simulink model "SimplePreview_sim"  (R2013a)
settings: Solver=ode45  StartTime=0.0  StopTime=60  RelTol=1e-3
undefined symbols (not defined in the file or in its folder): A, B, Bw, C_all, x0

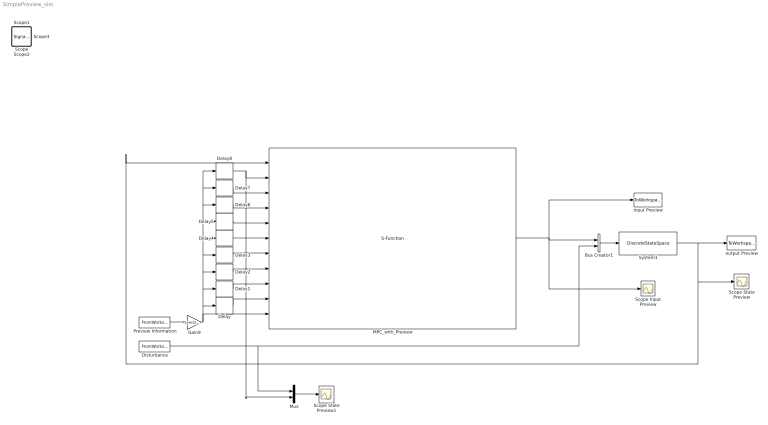
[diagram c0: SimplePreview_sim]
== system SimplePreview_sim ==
  Bus Creator1 : BusCreator  Inputs=2
  Delay : Delay  DelayLength=1  InitialCondition=0  SampleTime=1
  Delay1 : Delay  InitialCondition=0  SampleTime=1
  Delay2 : Delay  DelayLength=3  InitialCondition=0  SampleTime=1
  Delay3 : Delay  DelayLength=4  InitialCondition=0  SampleTime=1
  Delay4 : Delay  DelayLength=5  InitialCondition=0  SampleTime=1
  Delay5 : Delay  DelayLength=6  InitialCondition=0  SampleTime=1
  Delay6 : Delay  DelayLength=7  InitialCondition=0  SampleTime=1
  Delay7 : Delay  DelayLength=8  InitialCondition=0  SampleTime=1
  Delay8 : Delay  DelayLength=9  InitialCondition=0  SampleTime=1
  Disturbance : FromWorkspace  VariableName=[time, Road]  SampleTime=0
  Gain9 : Gain  Gain=ones(2,1)
  Input Preview : ToWorkspace  VariableName=input_u_pre  SampleTime=-1  SaveFormat=Timeseries
  MPC_with_Preview : S-Function  FunctionName=MPC_with_Preview_simulinkBlock  EnableBusSupport=off
  Mux : Mux  Inputs=2
  Preview Information : FromWorkspace  VariableName=[time, Pre]  SampleTime=0
  Scope Input Preview : Scope
  Scope State Preview : Scope
  Scope State Preview1 : Scope
  System1 : DiscreteStateSpace  A=A  B=[B, Bw]  C=C_all  D=zeros(2,2)  X0=x0
  output Preview : ToWorkspace  VariableName=state_x_pre  SampleTime=-1  SaveFormat=Timeseries
  Scope : SignalViewerScope  IOType=viewer  ZoomMode=yonly  RefreshTime=0.035000
  Scope1 : SignalViewerScope  IOType=viewer  RefreshTime=0.035000
  Scope2 : SignalViewerScope  IOType=viewer  RefreshTime=0.035000
  Scope3 : SignalViewerScope  IOType=viewer  RefreshTime=0.035000
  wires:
  MPC_with_Preview/1 -> Scope Input Preview/1, Bus Creator1/1, Input Preview/1
  System1/1 -> MPC_with_Preview/1, Scope State Preview/1, output Preview/1
  Bus Creator1/1 -> System1/1
  Delay8/1 -> Mux/2, MPC_with_Preview/2
  Delay7/1 -> MPC_with_Preview/3
  Delay6/1 -> MPC_with_Preview/4
  Delay5/1 -> MPC_with_Preview/5
  Delay4/1 -> MPC_with_Preview/6
  Delay3/1 -> MPC_with_Preview/7
  Delay2/1 -> MPC_with_Preview/8
  Delay1/1 -> MPC_with_Preview/9
  Delay/1 -> MPC_with_Preview/10
  Preview Information/1 -> Gain9/1
  Mux/1 -> Scope State Preview1/1
  Gain9/1 -> MPC_with_Preview/11, Delay/1, Delay1/1, Delay2/1, Delay3/1, Delay4/1, Delay5/1, Delay6/1, Delay7/1, Delay8/1
  Disturbance/1 -> Mux/1, Bus Creator1/2
